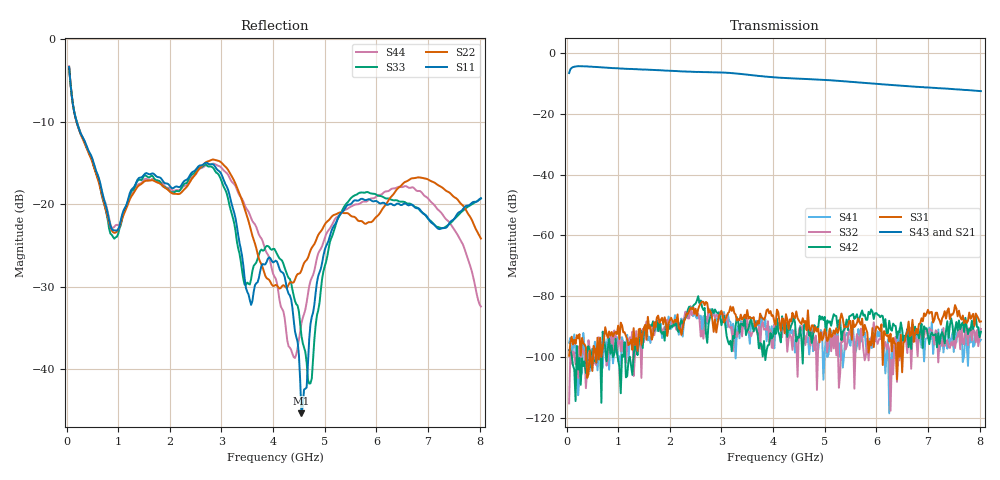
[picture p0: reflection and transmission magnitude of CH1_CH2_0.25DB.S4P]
!Agilent Technologies,E5071C,MY46316741,A.11.02
!Date: Thu May 28 14:24:59 2026
!Data & Calibration Information:
!1:CH1 INPUT 2:CH1 OUTPUT 3:CH2 INPUT 4:CH2 OUTPUT
!Freq	S11:SOLT4(ON)	S12:SOLT4(ON)	S13:SOLT4(ON)	S14:SOLT4(ON)
!	S21:SOLT4(ON)	S22:SOLT4(ON)	S23:SOLT4(ON)	S24:SOLT4(ON)
!	S31:SOLT4(ON)	S32:SOLT4(ON)	S33:SOLT4(ON)	S34:SOLT4(ON)
!	S41:SOLT4(ON)	S42:SOLT4(ON)	S43:SOLT4(ON)	S44:SOLT4(ON)
!PortZ  Port1:50+j0  Port2:50+j0  Port3:50+j0  Port4:50+j0
!Above PortZ is port z conversion or system Z0 setting when saving the data.
!When reading, reference impedance value at option line is always used.
# Hz S dB R 50
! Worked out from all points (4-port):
!   320 points, 50 MHz to 8.025 GHz, reference 50 ohm
!   strongest paths, dB at 50 MHz, 2.05 GHz, 4.05 GHz, 6.05 GHz, 8.025 GHz:
!     S43: -6.7, -6.0, -8.1, -10.3, -12.6
!     S21: -6.8, -6.1, -8.2, -10.3, -12.6
!     S31: -99.5, -88.0, -89.3, -90.7, -88.3
!     S42: -97.7, -90.0, -92.4, -86.2, -91.6
!     S32: -115.2, -88.1, -90.9, -94.1, -90.7
!     S41: -95.2, -89.9, -88.8, -93.2, -94.3
!   lowest |S11| = -45.3 dB at 4.55 GHz (marker M1), VSWR 1.01, Z = 50 - j0.54 ohm
!   |S11| at or under -10 dB: 196.9 MHz to end of sweep
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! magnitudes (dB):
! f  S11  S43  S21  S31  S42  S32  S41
! 50 MHz  -3.4  -6.7  -6.8  -99.5  -97.7  -115.2  -95.2
! 900 MHz  -23.1  -5.0  -5.2  -93.2  -100.0  -97.8  -102.0
! 2.85 GHz  -15.2  -6.4  -6.6  -91.7  -85.5  -85.7  -84.8
! 4.225 GHz  -28.8  -8.3  -8.4  -92.1  -89.8  -90.7  -91.3
! 4.55 GHz  -45.3  -8.5  -8.6  -89.1  -94.1  -90.7  -91.1
! 5.425 GHz  -20.2  -9.4  -9.5  -90.0  -87.6  -96.5  -92.1
! 8.025 GHz  -19.3  -12.6  -12.6  -88.3  -91.6  -90.7  -94.3
